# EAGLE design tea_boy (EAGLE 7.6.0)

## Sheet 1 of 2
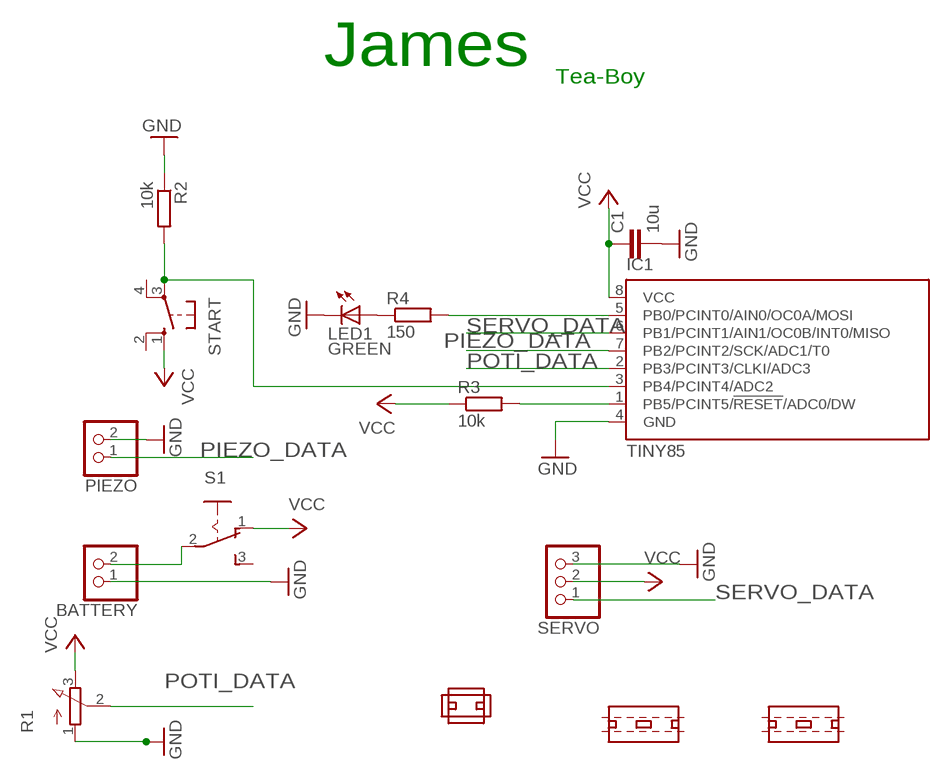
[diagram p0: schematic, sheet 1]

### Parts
BATTERY  PINHD-1X2  [1X02]
C1  10u  C-EU025-024X044  [C025-024X044]
IC1  TINY85  TINY13-20PU  [DIL08]
LED1  GREEN  LED5MM  [LED5MM]
PIEZO  PINHD-1X2  [1X02]
R1  3RP/1610N  [3RP/1610N]
R2  10k  R-EU_0207/10  [0207/10]
R3  10k  R-EU_0207/10  [0207/10]
R4  150  R-EU_0207/10  [0207/10]
S1  M251  [M251]
SERVO  PINHD-1X3  [1X03]
START  10-XX  [B3F-10XX]
U$1  MAJA_CLAMP  [MAJA_CLAMP_PACKAGE]
U$2  MAJA_CLAMP_2  [MAJA_CLAMP_PACKAGE_2]
U$3  MAJA_CLAMP_2  [MAJA_CLAMP_PACKAGE_2]

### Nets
GND: BATTERY.1 C1.2 IC1.4(GND) LED1.K(C) PIEZO.2 R1.1(A) R2.1 SERVO.3 ; also sheet 2
N$1: LED1.A R4.1
N$2: IC1.3(PB4/PCINT4/ADC2) R2.2 START.3(P)
N$3: IC1.5(PB0/PCINT0/AIN0/OC0A/MOSI) R4.2
N$4: BATTERY.2 S1.2(P)
N$5: IC1.1(PB5/PCINT5/!RESET!/ADC0/DW) R3.2
PIEZO_DATA: IC1.7(PB2/PCINT2/SCK/ADC1/T0) PIEZO.1
POTI_DATA: IC1.2(PB3/PCINT3/CLKI/ADC3) R1.2(S)
SERVO_DATA: IC1.6(PB1/PCINT1/AIN1/OC0B/INT0/MISO) SERVO.1
VCC: C1.1 IC1.8(VCC) R1.3(E) R3.1 S1.1(O) SERVO.2 START.1(S) ; also sheet 2
Unconnected: S1.3(S) START.2(S1) START.4(P1)

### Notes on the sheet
- James
- Tea-Boy

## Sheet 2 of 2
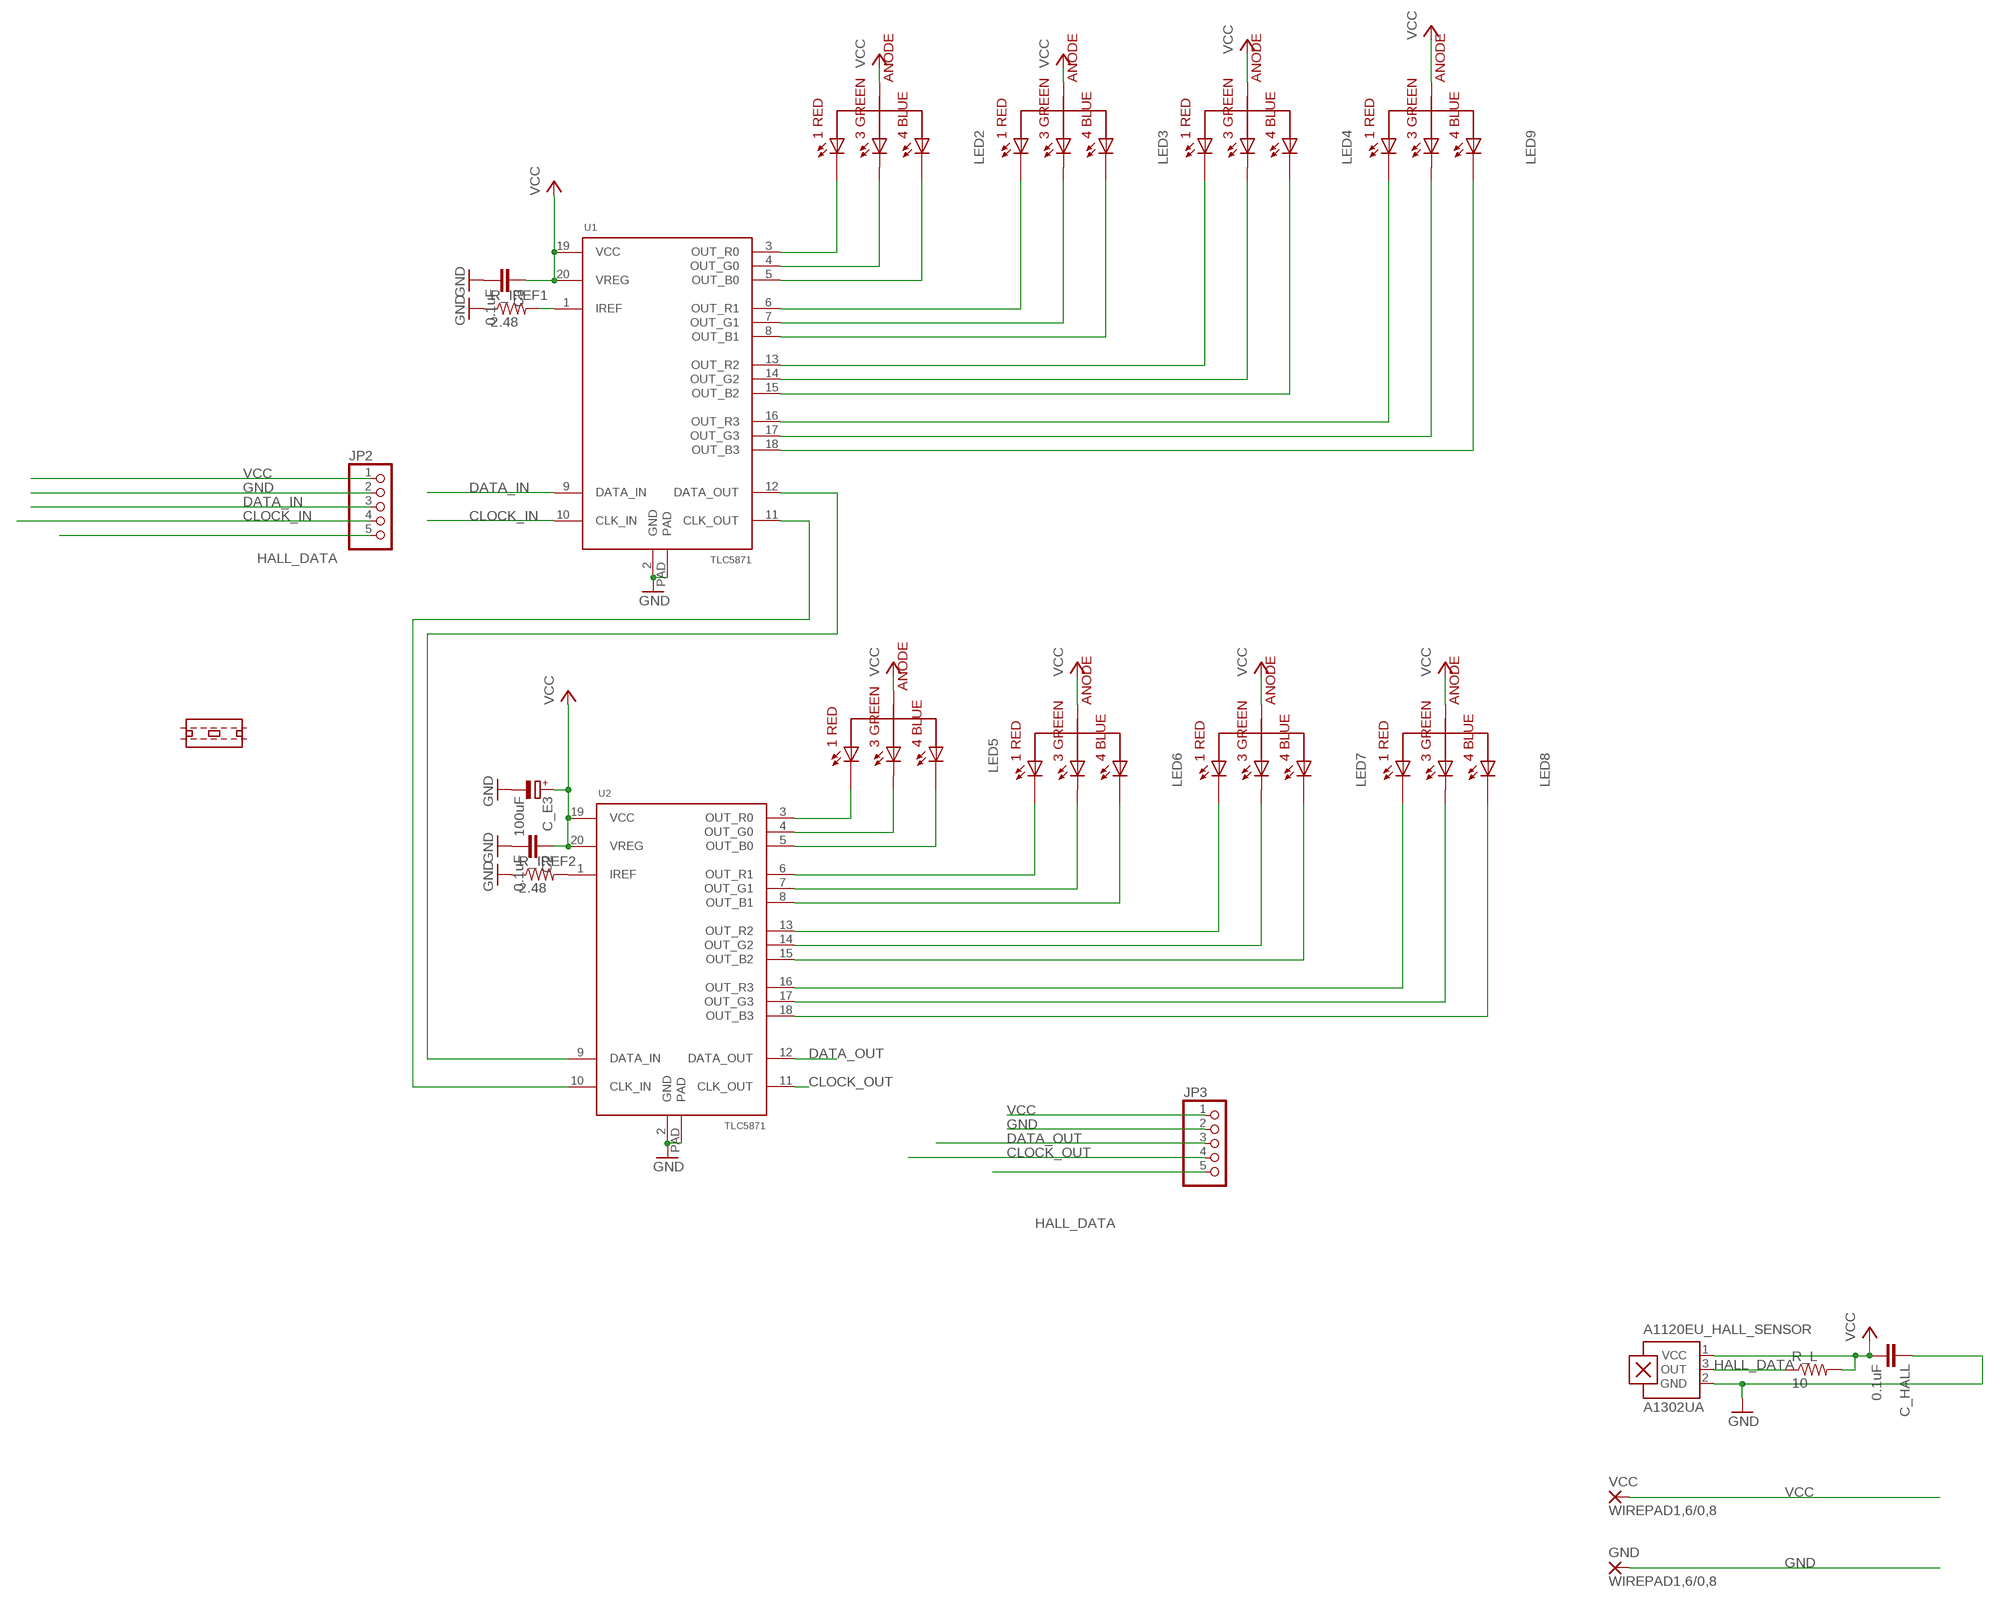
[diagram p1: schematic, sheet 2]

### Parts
A1120EU_HALL_SENSOR  A1302UA  [SIP3-UA]
C2  0.1uF  C-EUC0805  [C0805]
C3  0.1uF  C-EUC0805  [C0805]
C_E3  100uF  CPOL-EUE2.5-6  [E2,5-6]
C_HALL  0.1uF  C-EUC0805  [C0805]
GND  WIREPAD1,6/0,8  [1,6/0,8]
JP2  PINHD-1X55X2MM  [1_05X2MM]
JP3  PINHD-1X55X2MM  [1_05X2MM]
LED2  RGBLED_HOLE  [RGBLED5MM_HOLE]
LED3  RGBLED_HOLE  [RGBLED5MM_HOLE]
LED4  RGBLED_HOLE  [RGBLED5MM_HOLE]
LED5  RGBLED_HOLE  [RGBLED5MM_HOLE]
LED6  RGBLED_HOLE  [RGBLED5MM_HOLE]
LED7  RGBLED_HOLE  [RGBLED5MM_HOLE]
LED8  RGBLED_HOLE  [RGBLED5MM_HOLE]
LED9  RGBLED_HOLE  [RGBLED5MM_HOLE]
R_IREF1  2.48  R-US_M0805  [M0805]
R_IREF2  2.48  R-US_M0805  [M0805]
R_L  10  R-US_M0805  [M0805]
U1  TLC5971  [R-PDSO-G20]
U2  TLC5971  [R-PDSO-G20]
U$4  MAJA_CLAMP_2  [MAJA_CLAMP_PACKAGE_2]
VCC  WIREPAD1,6/0,8  [1,6/0,8]

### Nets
CLOCK_IN: JP2.4 U1.10(CLK_IN)
CLOCK_OUT: JP3.4 U2.11(CLK_OUT)
DATA_IN: JP2.3 U1.9(DATA_IN)
DATA_OUT: JP3.3 U2.12(DATA_OUT)
GND: A1120EU_HALL_SENSOR.2(GND) C2.2 C3.2 C_E3.- C_HALL.1 GND.1(P) JP2.2 JP3.2 R_IREF1.1 R_IREF2.1 U1.2(GND) U1.PAD U2.2(GND) U2.PAD ; also sheet 1
HALL_DATA: A1120EU_HALL_SENSOR.3(OUT) JP2.5 JP3.5 R_L.1
N$15: R_IREF2.2 U2.1(IREF)
N$16: LED5.A1_RED U2.3(OUT_R0)
N$17: LED5.A3_GREEN U2.4(OUT_G0)
N$18: LED5.A4_BLUE U2.5(OUT_B0)
N$19: LED6.A1_RED U2.6(OUT_R1)
N$20: LED6.A3_GREEN U2.7(OUT_G1)
N$21: LED6.A4_BLUE U2.8(OUT_B1)
N$22: LED7.A1_RED U2.13(OUT_R2)
N$23: LED7.A3_GREEN U2.14(OUT_G2)
N$24: LED7.A4_BLUE U2.15(OUT_B2)
N$25: LED8.A1_RED U2.16(OUT_R3)
N$26: LED8.A3_GREEN U2.17(OUT_G3)
N$27: LED8.A4_BLUE U2.18(OUT_B3)
N$28: U1.12(DATA_OUT) U2.9(DATA_IN)
N$29: U1.11(CLK_OUT) U2.10(CLK_IN)
N$30: R_IREF1.2 U1.1(IREF)
N$33: LED2.A1_RED U1.3(OUT_R0)
N$34: LED2.A3_GREEN U1.4(OUT_G0)
N$35: LED2.A4_BLUE U1.5(OUT_B0)
N$36: LED3.A1_RED U1.6(OUT_R1)
N$37: LED3.A3_GREEN U1.7(OUT_G1)
N$38: LED3.A4_BLUE U1.8(OUT_B1)
N$39: LED4.A1_RED U1.13(OUT_R2)
N$40: LED4.A3_GREEN U1.14(OUT_G2)
N$41: LED4.A4_BLUE U1.15(OUT_B2)
N$42: LED9.A1_RED U1.16(OUT_R3)
N$43: LED9.A3_GREEN U1.17(OUT_G3)
N$44: LED9.A4_BLUE U1.18(OUT_B3)
VCC: A1120EU_HALL_SENSOR.1(VCC) C2.1 C3.1 C_E3.+ C_HALL.2 JP2.1 JP3.1 LED2.A2_VCC(A2_ANODE) LED3.A2_VCC(A2_ANODE) LED4.A2_VCC(A2_ANODE) LED5.A2_VCC(A2_ANODE) LED6.A2_VCC(A2_ANODE) LED7.A2_VCC(A2_ANODE) LED8.A2_VCC(A2_ANODE) LED9.A2_VCC(A2_ANODE) R_L.2 U1.19(VCC) U1.20(VREG) U2.19(VCC) U2.20(VREG) VCC.1(P) ; also sheet 1

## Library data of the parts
A1120EU_HALL_SENSOR = allegro:A13*?: Linear Hall Effect Sensor ICs Continuous-Time Ratiometric High-Temperature Operation Programmable Linear with Analog Output A1302 -Replacement- UGN3503 Source: http://www.allegromicro.com/en/Products/Part_Numbers/1301/1301.pdf http://www.allegromicro.com/en/Products/Part_Numbers/1321/1321.pdf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; MF: ALLEGRO MICROSYSTEMS, INC.; MPN: A1302EUA-T; OC_FARNELL: 1521708; OC_NEWARK: 31K6639
BATTERY PIEZO = pinhead:PINHD-1X2: PIN HEADER
C1 = resistor:C-EU: CAPACITOR, European symbol
C2 C3 C_HALL = rcl:C-EU: CAPACITOR, European symbol
C_E3 = rcl:CPOL-EU: POLARIZED CAPACITOR, European symbol
GND VCC = wirepad:WIREPAD: Wire PAD connect wire on PCB
IC1 = atmel:TINY13: 8-bit AVR Microcontroller with 1K Bytes In-System Programmable Flash Source: http://www.atmel.com/dyn/resources/prod_documents/2535S.pdf; MPN: ATTINY13-20PU; OC_FARNELL: 9171550; OC_NEWARK: 96K6521
JP2 JP3 = pinhead:PINHD-1X5: PIN HEADER
LED1 = led:LED: LED
LED2-LED9 = rgb_led:RGBLED_HOLE
R1 = pot:3RP/1610N: 16mm Potentiometer one level Source: http://www.alphapotentiometers.net/html/16mm_pot_2.html
R2-R4 = resistor:R-EU_: RESISTOR, European symbol
R_IREF1 R_IREF2 R_L = rcl:R-US_: RESISTOR, American symbol
S1 = switch:M251: SLIDING SWITCH Mors, distributor Buerklin, 11G702
SERVO = pinhead:PINHD-1X3: PIN HEADER
START = switch-omron:10-XX: OMRON SWITCH; MPN: B3F-1000; OC_FARNELL: 176432; OC_NEWARK: 36M3542
U1 U2 = TLC5971:TLC5971: RGB LED Driver with PWM, Constant current, RGB Color aware.; AVAILABILITY: Unavailable; DESCRIPTION: 12-Channel 16-Bit ES-PWM RGB LED Driver with 3.3V Linear Regulator; MF: Texas Instruments; MP: TLC5971; PACKAGE: None; PRICE: None
U$1 = single_clamp:MAJA_CLAMP
U$2-U$4 = single_clamp:MAJA_CLAMP_2

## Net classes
1 a: width 0.203 mm, drill 0.305 mm, clearance 0.203 mm

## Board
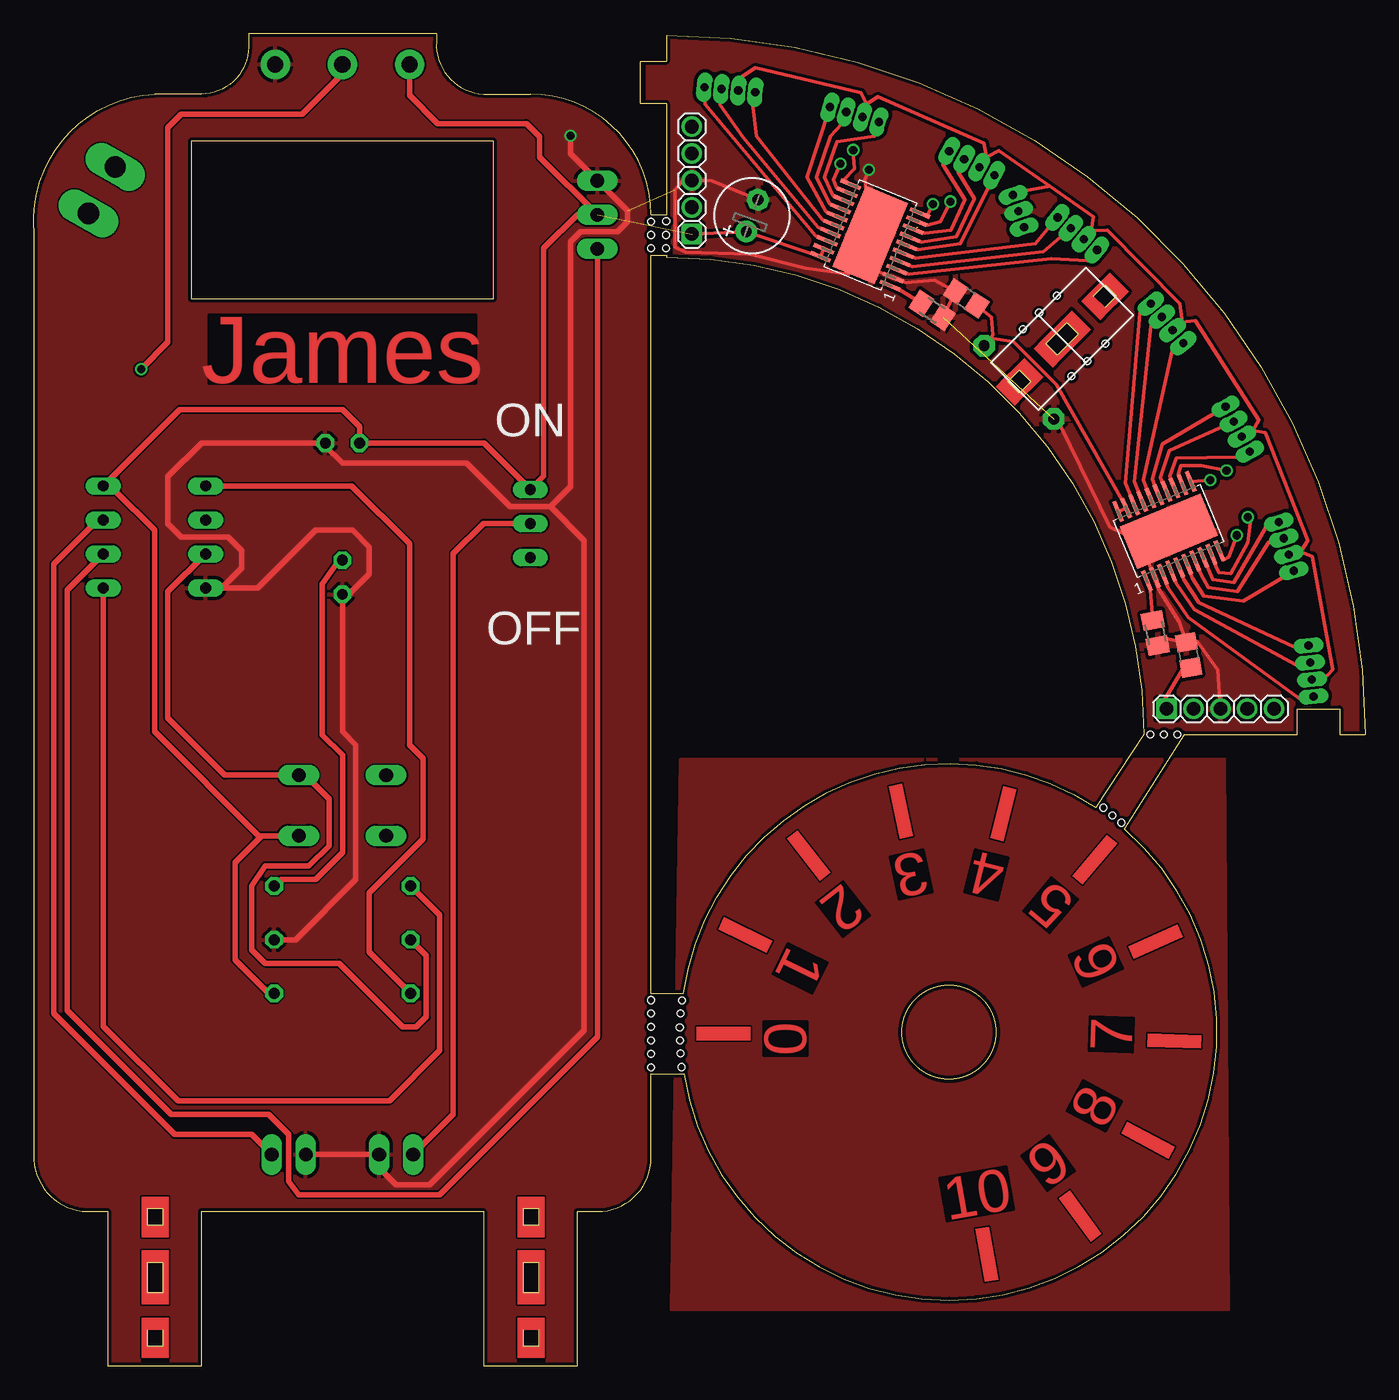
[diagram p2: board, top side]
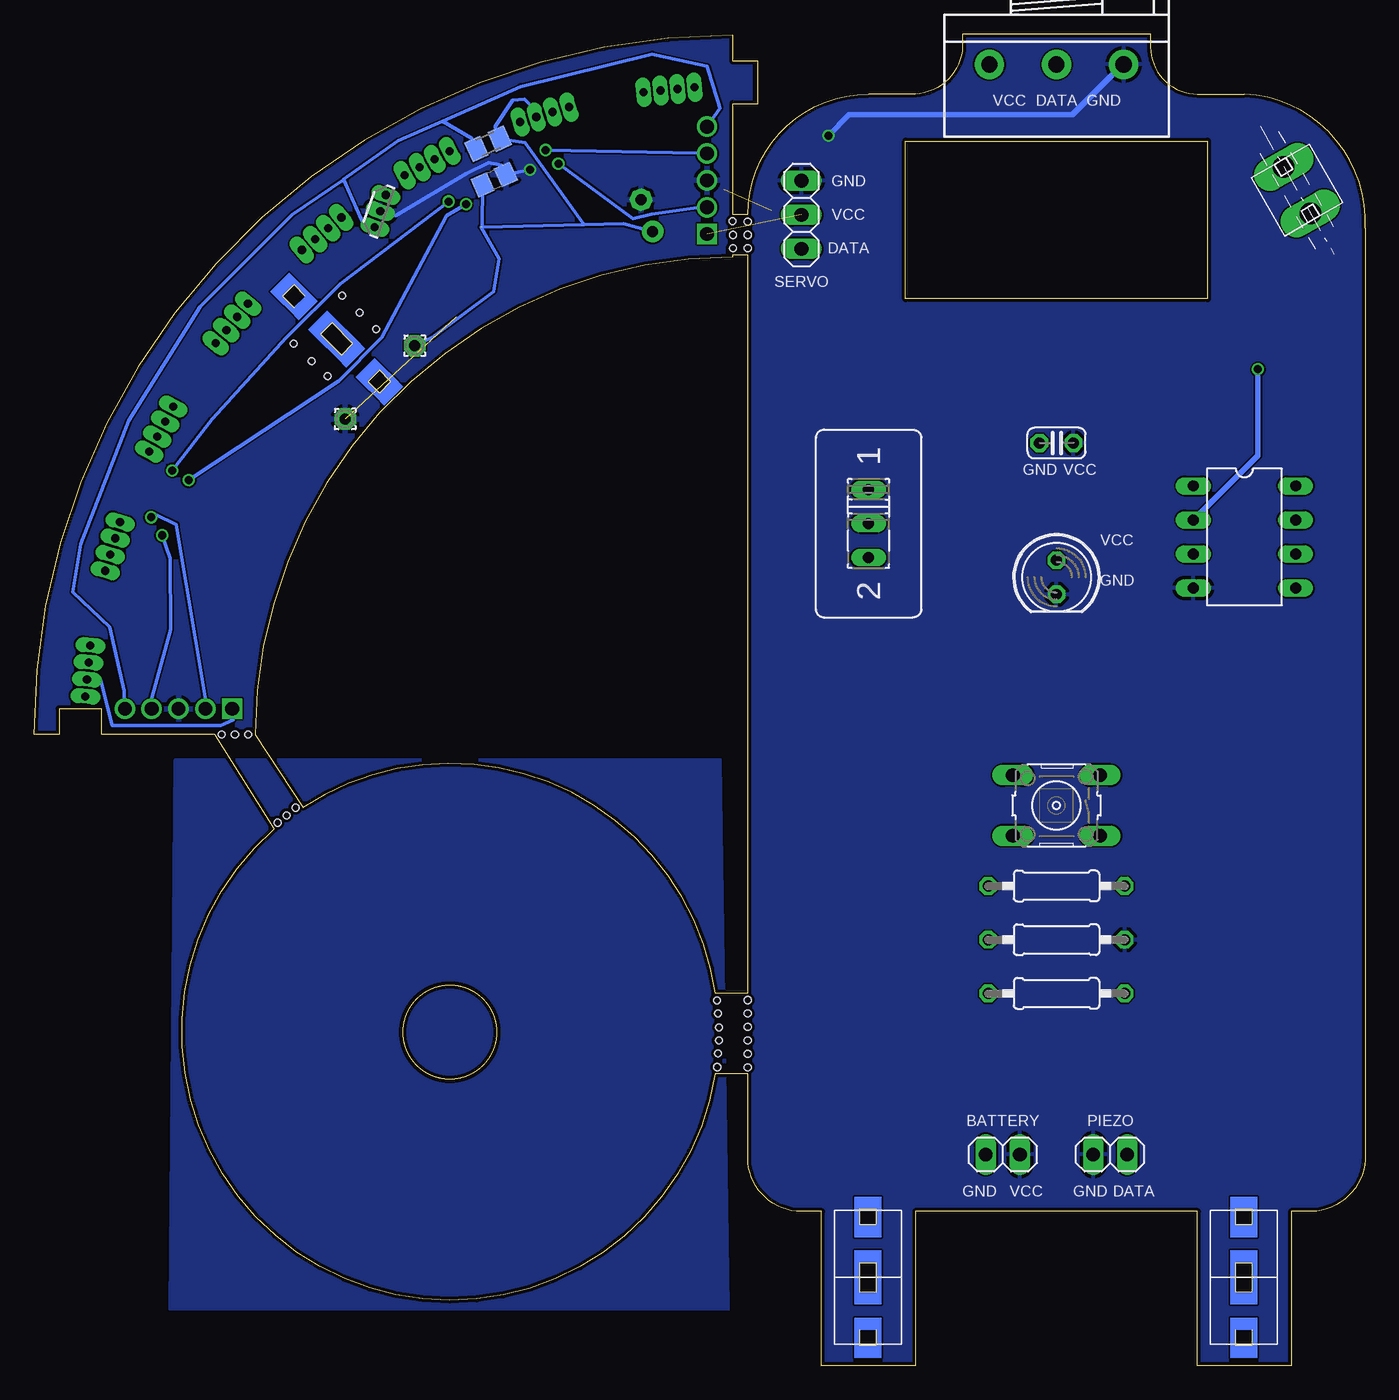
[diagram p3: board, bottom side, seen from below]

Size 99.21 x 99.25 mm. Coordinates in mm from the lower left corner, seen from the top.
Outline: 4.01,11.5 5.51,11.5 5.51,0 12.51,0 12.51,11.5 33.51,11.5 33.51,0 40.51,0 40.51,11.5 42.01,11.5 arc90 46.01,15.5 46.01,21.75 48.44,21.75 arc220 81.27,39.98 85.71,47.04 94.13,47.04 94.13,48.95 97.3,48.95 97.3,47.04 99.21,47.04 arc90 47.14,99.11 47.14,97.2 45.23,97.2 45.23,94.03 47.14,94.03 47.14,85.75 46.01,85.75 arc90 37.01,94.75 33.51,94.75 arc-90 30.01,98.65 30.01,99.25 16.01,99.25 16.01,98.25 arc-90 12.51,94.75 9.01,94.75 arc90 0.01,84.75 0.01,15.75 arc90 4.01,11.5
Outline: 11.76,79.5 34.26,79.5 34.26,91.25 11.76,91.25 11.76,79.5
Outline: 46.01,27.75 46.01,82.75 47.14,82.75 47.14,82.6 arc-90 82.7,47.04 79.13,41.62 arc115 48.41,27.75 46.01,27.75
Outline: circle at 68.2,24.86 radius 3.5
Copper layers (1*16): Top 0.035mm / dielectric 1.5mm / Bottom 0.035mm
Design rules "designrules_dirtypcbs": minimum track width 5mil, minimum drill 12mil, track to track 5mil, track to pad 5mil, pad to pad 5mil, via to via 5mil, smd to smd 0mil, copper to edge 10mil, drill to drill 10mil, minimum pad ring 10mil, minimum via ring 6mil, stop-mask expansion 2mil, vias tented up to drill 25mil, thermal gap 10mil
Holes 0.5 mm at 46.01,85.25 47.13,85.26 47.11,84.25 46.01,84.25 46.01,83.25 47.11,83.25 46.01,27.25 46.01,26.25 46.01,25.25 46.01,24.25 46.01,23.25 46.01,22.25 48.3,27.25 48.21,26.25 48.13,25.23 48.16,24.25 48.21,23.27 48.28,22.26 73.7,77.24 74.91,78.45 76.22,79.74 77.31,73.72 78.51,74.85 79.84,76.15 81.03,40.47 79.69,41.58 80.36,41.01 83.21,47.05 84.21,47.05 85.21,47.05
tRestrict: 4 lines

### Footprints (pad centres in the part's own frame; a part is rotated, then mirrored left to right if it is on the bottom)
SIP3-UA = drill 0.6 pad 0.7 long: 1 -1.27,0; 2 0,0; 3 1.27,0
1X02 = drill 1.016 long: 1 -1.27,0; 2 1.27,0
C025-024X044 = drill 0.813 octagon: 1 -1.27,0; 2 1.27,0
C0805 = smd 1.3 x 1.5: 1 -0.95,0; 2 0.95,0
E2,5-6 = drill 0.813 pad 1.6: + -1.27,0 | drill 0.813 pad 1.6 octagon: - 1.27,0
1,6/0,8 = drill 0.813 pad 1.6 octagon: 1 0,0
DIL08 = drill 0.813 long: 1 -3.81,-3.81; 2 -1.27,-3.81; 3 1.27,-3.81; 4 3.81,-3.81; 5 3.81,3.81; 6 1.27,3.81; 7 -1.27,3.81; 8 -3.81,3.81
1_05X2MM = drill 1.016 pad 1.3 square: 1 -4,0 | drill 1.016 pad 1.3: 2 0,0; 3 -2,0; 4 2,0; 5 4,0
LED5MM = drill 0.813 octagon: A -1.27,0; K 1.27,0
RGBLED5MM_HOLE = drill 0.61 pad 0.711 long: A1_RED 1.905,0; A2_VCC 0.635,0; A3_GREEN -0.635,0; A4_BLUE -1.905,0
3RP/1610N = drill 1.2 pad 2.184: 1 -5,0; 2 0,0; 3 5,0
0207/10 = drill 0.813 octagon: 1 -5.08,0; 2 5.08,0
M0805 = smd 1.3 x 1.6: 1 -0.95,0; 2 0.95,0
M251 = drill 0.813 long: 1 -2.54,0; 2 0,0; 3 2.54,0
1X03 = drill 1.016 long: 1 -2.54,0; 2 0,0; 3 2.54,0
B3F-10XX = drill 1.016 long: 1 -3.251,2.261; 2 3.251,2.261; 3 -3.251,-2.261; 4 3.251,-2.261
R-PDSO-G20 = smd 0.3 x 1.6: 1 -2.925,-2.8; 2 -2.275,-2.8; 3 -1.625,-2.8; 4 -0.975,-2.8; 5 -0.325,-2.8; 6 0.325,-2.8; 7 0.975,-2.8; 8 1.625,-2.8; 9 2.275,-2.8; 10 2.925,-2.8; 11 2.925,2.8; 12 2.275,2.8; 13 1.625,2.8; 14 0.975,2.8; 15 0.325,2.8; 16 -0.325,2.8; 17 -0.975,2.8; 18 -1.625,2.8; 19 -2.275,2.8; 20 -2.925,2.8 | smd 6.5 x 3.4: PAD 0,0
MAJA_CLAMP_PACKAGE = drill 1.58 pad 2.184 long: P$1 0.5,2.5; P$2 4.5,2.5

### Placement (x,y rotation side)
A1120EU_HALL_SENSOR  73.37,86.03 251 bottom
BATTERY  27.01,15.75 180 bottom
C1  23.01,68.75 0 bottom
C2  69.47,79.52 146.8 top
C3  86.03,52.96 100 top
C_E3  53.52,85.69 70 top
C_HALL  64.89,88.37 204 bottom
GND  75.99,70.53 0 bottom
IC1  9.01,61.75 270 bottom
JP2  88.41,48.95 0 top
JP3  49.04,88.31 90 top
LED1  23.01,58.75 270 bottom
LED2  95.16,51.77 275.6 top
LED3  93.32,61.05 286.9 top
LED4  89.7,69.79 298.1 top
LED5  77.75,84.35 320.6 top
LED6  69.89,89.6 331.9 top
LED7  61.14,93.22 343.1 top
LED8  51.87,95.07 354.4 top
LED9  84.44,77.66 309.4 top
PIEZO  19.01,15.75 180 bottom
R1  23.01,96.95 180 bottom
R2  23.01,31.75 180 bottom
R3  23.01,27.75 180 bottom
R4  23.01,35.75 180 bottom
R_IREF1  83.56,54.6 101.3 top
R_IREF2  66.94,78.64 147 top
R_L  65.35,91.03 24 bottom
S1  37.01,62.75 270 bottom
SERVO  42.01,85.75 90 bottom
START  23.01,41.75 180 bottom
U1  84.56,62.19 22.5 top
U2  62.32,84.25 67.5 top
U$1  8.51,88.5 300 bottom
U$2  9.06,6.6 90 bottom
U$3  37.06,6.6 90 bottom
U$4  76.63,76.5 225 top
VCC  70.81,76 0 bottom

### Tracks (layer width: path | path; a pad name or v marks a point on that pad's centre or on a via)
CLOCK_IN  (via drill 0.6)
  Top 0.254: v89.63,61.87 89.05,60.25 88.61,60.02 U1.10
  Bottom 0.254: JP2.4 90.39,49.71 88.99,54.84 89.02,60.15 v89.63,61.87
CLOCK_OUT  (via drill 0.6)
  Top 0.254: v61.05,90.58 61.16,89.18 60.37,88.37 U2.11
  Bottom 0.254: JP3.4 49.73,90.35 v61.05,90.58
DATA_IN  (via drill 0.6)
  Top 0.254: v90.44,63.22 90.65,62.79 90.47,61.34 89.17,59.03 88.28,59.1 88.05,59.59 U1.9
  Bottom 0.254: JP2.3 86.38,49.6 88.56,62.69 90.11,63.42 v90.44,63.22
DATA_OUT  (via drill 0.6)
  Top 0.254: v60.11,89.56 59.58,88.37 59.81,87.78 U2.12
  Bottom 0.254: JP3.3 49.8,86.28 53.16,85.8 54.55,85.44 v60.11,89.56
GND  (via drill 0.6)  (2 unrouted)
  Top 0.254: R_IREF2.1 C2.2 67.1,80.9 64.97,80.69 U2.2 62.76,81.58 U2.PAD | C_E3.- 50.49,88.29 JP3.2 48.35,88.26 47.76,87.61 47.76,83.35 48.56,82.96 53.38,82.8 57.5,81.79 60.75,81.33 U2.PAD | R_IREF1.1 84.35,54.18 C3.2 | C3.2 86.68,53.95 88.23,51.84 JP2.2 | C3.2 85.36,55.4 83.79,57.91 U1.2 83.05,59.89 83.67,60.83 | 83.67,60.83 U1.PAD | GND.1 76.47,70.05 80.18,62.48 83.67,60.83 | v62.22,89.1 61.94,88.37 U2.PAD
  Top 0.406: R2.1 19.51,31.75 24.01,36.25 24.01,46.25 23.01,47.25 LED1.K 23.24,57.25 23.26,57.25 25.01,59 25.01,61 23.76,62.25 21.01,62.25 16.7,57.94 14.01,57.94 | IC1.4 14.01,57.94 | 14.01,57.94 15.51,59.44 15.51,60.75 14.51,61.75 11.01,61.75 10.01,62.75 10.01,66.25 12.51,68.75 C1.2 21.74,68.52 23.01,67.25 32.26,67.25 35.51,64 38.51,64 | 38.51,64 40.01,65.5 40.01,83.75 40.76,84.5 43.51,84.5 44.26,85.25 44.26,86.04 SERVO.3 40.01,90.29 v40.01,91.65 | 38.51,64 41.01,61.5 41.01,25 29.51,13.5 27.01,13.5 26.01,14.5 26.01,15.25 25.74,15.52 BATTERY.1 PIEZO.2
  Bottom 0.254: A1120EU_HALL_SENSOR.2 72.23,85.7 66.97,88.82 65.3,89.64 64.33,89.43 C_HALL.1 v62.22,89.1
  Bottom 0.406: R1.1 18.06,96.95 21.81,93.2 38.46,93.2 v40.01,91.65
  pour Top (isolate 0.1): -0.49,99.25 -0.49,-0.75 46.01,-0.75 45.91,99.25
  pour Bottom: 0.01,99.25 0.01,-0.75 46.01,-0.75 46.01,99.25
  pour Top (isolate 0.254): 45.83,99.11 99.21,97.84 99.21,47.04 45.83,47.04
  pour Bottom: 45.83,99.11 99.21,97.84 99.21,47.04 45.83,47.04
HALL_DATA
  Bottom 0.254: 68.73,92.73 72.05,91.26 76.12,88.39 74.77,85.34 A1120EU_HALL_SENSOR.3 74.64,85.14 76.09,88.37 79.93,85.78 86.81,78.92 92.12,70.41 95.67,61.21 96.28,57.63 93.54,55.04 92.45,50.29 JP2.5 | 68.73,92.73 62.93,95.3 53.13,97.71 49.04,96.8 48.08,93.67 JP3.5 | R_L.1 66.57,91.44 68.73,92.73
N$1
  Top 0.406: LED1.A 22.78,60.02 21.51,58.25 21.51,47 23.01,45.5 23.01,38.25 21.01,36.25 18.43,36.25 R4.1
N$2
  Top 0.406: IC1.3 10.01,57.67 10.01,48.25 14.24,44.01 START.3 20.24,44.01 22.01,42.25 22.01,38.75 20.51,37.25 17.26,37.25 16.26,35.75 16.26,31 17.26,30 22.76,30 27.51,25.25 28.51,25.25 29.26,26 29.26,30.58 R2.2
N$3
  Top 0.406: IC1.5 5.2,25.31 10.76,19.75 26.51,19.75 30.26,23.5 30.26,33.58 R4.2
N$4
  Top 0.406: S1.2 33.51,62.75 31.26,60.5 31.26,18.73 BATTERY.2
N$5
  Top 0.406: IC1.1 23.7,65.56 28.01,61.25 28.01,46.25 29.01,45.25 29.01,39.25 25.01,35.25 25.01,30.83 R3.2
N$6
  pour Bottom: 48.11,45.15 47.51,4.25 89.01,4.25 88.61,45.15
  pour Top: 48.21,45.15 47.51,4.25 89.01,4.25 88.71,45.15
N$15
  Top 0.254: U2.1 64.51,80.16 R_IREF2.2
N$16
  Top 0.254: U2.3 65.19,81.33 75.81,82.47 78.5,82.32 LED5.A1_RED
N$17
  Top 0.254: U2.4 65.45,81.89 75.23,83.01 LED5.A3_GREEN
N$18
  Top 0.254: U2.5 65.68,82.52 74.64,83.59 LED5.A4_BLUE
N$19
  Top 0.254: LED6.A1_RED 69.03,83.62 65.88,83.16 U2.6
N$20
  Top 0.254: U2.7 66.13,83.72 68.73,84.12 70.07,86.94 68.85,88.97 LED6.A3_GREEN
N$21
  Top 0.254: U2.8 66.41,84.38 68.34,84.61 69.39,86.89 67.73,89.48 LED6.A4_BLUE
N$22
  Top 0.254: LED7.A1_RED 62.65,91.62 59.84,91.21 58.92,88.54 59.53,87.17 U2.13
N$23
  Top 0.254: U2.14 59.3,86.56 58.31,88.57 59.35,91.59 60.19,92.51 LED7.A3_GREEN
N$24
  Top 0.254: LED7.A4_BLUE 57.63,88.57 59.02,85.98 U2.15
N$25
  Top 0.254: U2.16 58.77,85.39 53.84,91.59 53.59,93.78 LED8.A1_RED
N$26
  Top 0.254: U2.17 58.44,84.81 52.85,91.52 51.12,93.95 LED8.A3_GREEN
N$27
  Top 0.254: LED8.A4_BLUE 50.03,94 58.24,84.2 U2.18
N$28  (via drill 0.6)
  Top 0.254: U2.9 66.57,84.99 67.56,85.24 v68.29,86.74 | U1.12 85.26,66.45 85.46,67.08 86.99,67.06 v88.87,66.7
  Bottom 0.254: v88.87,66.7 85.9,70.53 80.37,76.59 76.31,80.62 v68.29,86.74
N$29  (via drill 0.6)
  Top 0.254: U2.10 66.57,85.72 v67,86.54 | v87.65,65.99 U1.11
  Bottom 0.254: v67,86.54 68.45,85.67 73.29,76.58 76.47,73.38 v87.65,65.99
N$30
  Top 0.254: U1.1 83.18,57.81 R_IREF1.2
N$33
  Top 0.254: LED2.A1_RED 94.28,49.73 86.02,55.75 84.5,57.99 U1.3
N$34
  Top 0.254: LED2.A3_GREEN 94.05,52.22 86.45,56.34 85.11,58.29 U1.4
N$35
  Top 0.254: LED2.A4_BLUE 93.9,53.54 86.81,56.87 85.67,58.6 U1.5
N$36
  Top 0.254: LED3.A1_RED 90.11,57 87.17,57.35 86.33,58.67 U1.6
N$37
  Top 0.254: LED3.A3_GREEN 92.02,61.37 89.68,57.68 87.5,57.99 86.94,59 U1.7
N$38
  Top 0.254: LED3.A4_BLUE 91.81,62.51 89.4,58.34 87.83,58.57 U1.8
N$39
  Top 0.254: LED4.A1_RED 89.68,67.69 85.11,67.64 84.63,66.29 U1.13
N$40
  Top 0.254: LED4.A3_GREEN 84.6,68.2 83.94,66.17 U1.14
N$41
  Top 0.254: LED4.A4_BLUE 84.07,68.68 83.33,66.06 U1.15
N$42
  Top 0.254: LED9.A1_RED 84.78,75.51 82.67,65.99 U1.16
N$43
  Top 0.254: LED9.A3_GREEN 83.23,77.47 83.23,77.44 82.01,65.89 U1.17
N$44
  Top 0.254: LED9.A4_BLUE 82.39,78.43 81.32,65.76 U1.18
PIEZO_DATA
  Top 0.406: IC1.7 4.78,63.02 1.51,59.75 1.51,26.25 10.51,17.25 16.24,17.25 PIEZO.1
POTI_DATA  (via drill 0.6)
  Top 0.406: R1.2 23.01,96.25 20.01,93.25 11.01,93.25 10.01,92.25 10.01,76.25 v8.01,74.25
  Bottom 0.406: v8.01,74.25 8.01,67.83 IC1.2
SERVO_DATA
  Top 0.406: SERVO.1 42.01,24.5 30.26,12.75 19.76,12.75 19.01,13.75 19.01,17.25 17.51,18.75 10.26,18.75 2.51,26.5 2.51,57.79 IC1.6
VCC  (2 unrouted)
  Top 0.254: LED8.A2_VCC 52.57,95.94 53.79,96.7 61.64,94.84 62.07,93.95 LED7.A2_VCC 62.05,94 62.91,94.54 70.81,91.08 70.96,90.09 LED6.A2_VCC 71.06,90.07 71.93,90.53 75.71,87.86 | 75.71,87.86 78.94,85.6 78.81,84.58 LED5.A2_VCC 78.89,84.56 80,84.61 85.39,79.12 85.59,77.75 LED9.A2_VCC 85.51,77.75 86.53,77.88 91.28,70.46 90.82,69.67 LED4.A2_VCC 90.85,69.67 91.74,69.52 94.91,61.47 94.4,60.68 LED3.A2_VCC 94.35,60.68 95.27,60.3 96.79,51.89 96.11,51.13 LED2.A2_VCC | C2.1 71.34,78.13 71.47,76.78 71.29,76.57 | 71.29,76.57 VCC.1 | U2.19 U2.20 C_E3.+ JP3.1 | C3.1 85.59,51.84 84.32,49.71 JP2.1 | U1.20 U1.19 80.94,64.72 76.2,73.1 73,76.3 71.29,76.57 | A1120EU_HALL_SENSOR.1 73.88,87.55 75.71,87.86
  Top 0.406: START.1 17.01,39.49 | 17.01,39.49 16.77,39.49 9.01,47.25 9.01,62.25 6.01,65.25 5.51,65.25 IC1.8 10.89,71.25 23.01,71.25 24.28,69.98 C1.1 33.55,68.75 S1.1 38.01,66.29 38.01,83.25 40.51,85.75 SERVO.2 37.71,90.05 37.71,91.55 36.71,92.55 30.11,92.55 28.01,94.65 R1.3 | R3.1 17.51,27.75 15.01,30.25 15.01,37.49 17.01,39.49
  Bottom 0.254: C_HALL.2 65.78,84.83 58.19,85.02 | 58.19,85.02 55.26,85.09 C_E3.+ | 65.88,84.83 64.53,82.5 64.94,80.01 69.49,76.63 VCC.1 | JP2.1 84.35,48.11 85.28,47.71 93.34,47.73 93.73,49.16 94.21,51.08 LED2.A2_VCC | LED7.A2_VCC 61.92,93.6 62.62,94.36 63.52,94.27 64.81,92.33 R_L.2 62.6,91.11 58.19,85.02
(copper drawn outside any net)
  shapes: Top area x11

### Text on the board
Top: James | 3 | 4 | 2 | 5 | 6 | 1 | 0 | 7 | 8 | 9 | 10
tNames: ON | OFF
bNames: GND | DATA | VCC | GND | VCC | DATA | VCC | GND | VCC | GND | DATA | GND | VCC | GND
tStop: James | 3 | 4 | 2 | 5 | 6 | 1 | 0 | 7 | 8 | 9 | 10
